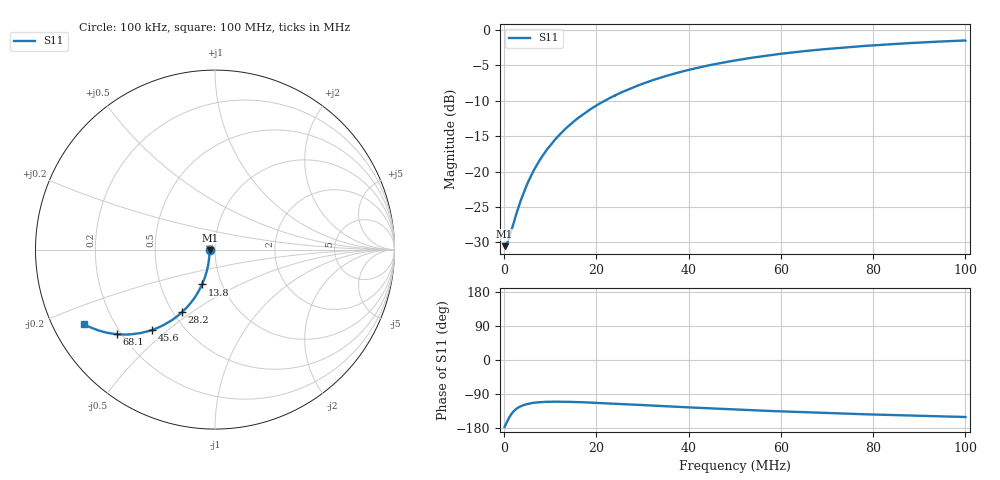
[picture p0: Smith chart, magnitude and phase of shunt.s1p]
# Hz S RI R 50.0
! written by SimSmith version 18.3h
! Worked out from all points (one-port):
!   1000 points, 100 kHz to 100 MHz, reference 50 ohm
!   lowest |S11| = -30.5 dB at 100 kHz (marker M1), VSWR 1.06, Z = 47.1 - j0.156 ohm
!   |S11| at or under -10 dB: start of sweep to 21.89 MHz
!   S11 on the Smith chart (normalised r, x): 100 kHz: 0.94, -0.00; 13.8 MHz: 0.81, -0.33; 28.2 MHz: 0.55, -0.46; 45.6 MHz: 0.33, -0.44; 68.1 MHz: 0.18, -0.36; 100 MHz: 0.10, -0.26
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100000  -0.0297 -0.00165
500000  -0.0298 -0.0075
1000000  -0.03 -0.0149
1500000  -0.0303 -0.0221
2900000  -0.032 -0.0426
3800000  -0.0334 -0.0559
4900000  -0.0358 -0.0718
6100000  -0.0386 -0.089
7400000  -0.0426 -0.1075
9000000  -0.0483 -0.13
1.07e7  -0.056 -0.1533
1.26e7  -0.0654 -0.1785
1.38e7  -0.0721 -0.1941
1.62e7  -0.0868 -0.2242
1.9e7  -0.1066 -0.2573
2.16e7  -0.1262 -0.2863
2.51e7  -0.1561 -0.3211
2.82e7  -0.1841 -0.349
3.26e7  -0.2257 -0.3829
3.76e7  -0.2745 -0.414
4.56e7  -0.3519 -0.4487
5.01e7  -0.3951 -0.4606
5.63e7  -0.451 -0.4703
6.26e7  -0.5036 -0.4732
6.81e7  -0.5461 -0.4714
7.51e7  -0.5952 -0.4642
8.76e7  -0.6695 -0.4432
1e8  -0.7271 -0.4136
